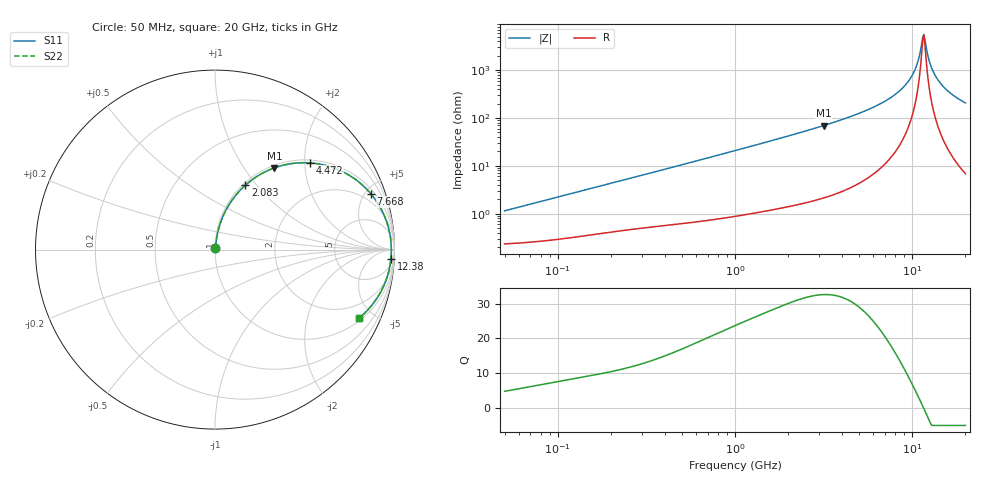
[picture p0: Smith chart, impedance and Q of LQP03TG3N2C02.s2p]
!Murata Part Number: LQP03TG3N2C02
!These Parameters are Measured in Series Mode Connection
!  o--[Z]--o
!Port1  Port2
!  o-------o
!Freq. Start=50[MHz] Stop=20[GHz], 401[Steps]
# Hz S RI R 50
!Freq.(Hz) S11(Real) S11(Imag) S21(Real) S21(Imag) S12(Real) S12(Imag) S22(Real) S22(Imag)
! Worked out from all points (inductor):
!   401 points, 50 MHz to 20 GHz, reference 50 ohm
!   read as one part in series: L = 3.56 nH near 51.52 MHz
!   highest Q = 32.6 at 3.169 GHz (marker M1), where L = 3.49 nH
!   self-resonance near 11.49 GHz
!   S11 on the Smith chart (normalised r, x): 50 MHz: 1.00, +0.02; 2.083 GHz: 1.03, +0.88; 4.472 GHz: 1.07, +2.13; 7.668 GHz: 1.31, +5.48; 12.38 GHz: 12, -33; 20 GHz: 1.14, -4.12
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5e7  0.00245 0.0112  0.9975 -0.0112  0.9975 -0.0112  0.00245 0.0112
1.364002e8  0.00425 0.0297  0.9957 -0.0297  0.9957 -0.0297  0.00425 0.0297
3.721004e8  0.0115 0.0772  0.9885 -0.0772  0.9885 -0.0772  0.0115 0.0772
1e9  0.049 0.1958  0.951 -0.1958  0.951 -0.1958  0.049 0.1958
2.083303e9  0.1695 0.3591  0.8305 -0.3591  0.8305 -0.3591  0.1695 0.3591
2.728004e9  0.2626 0.4248  0.7374 -0.4248  0.7374 -0.4248  0.2626 0.4248
3.168813e9  0.3306 0.4553  0.6694 -0.4553  0.6694 -0.4553  0.3306 0.4553
4.472136e9  0.5296 0.4831  0.4704 -0.4831  0.4704 -0.4831  0.5296 0.4831
5.944466e9  0.7184 0.4305  0.2816 -0.4305  0.2816 -0.4305  0.7184 0.4305
7.442007e9  0.8536 0.3276  0.1464 -0.3276  0.1464 -0.3276  0.8536 0.3276
7.668323e9  0.8691 0.3099  0.1309 -0.3099  0.1309 -0.3099  0.8691 0.3099
8.907419e9  0.9338 0.2098  0.0662 -0.2098  0.0662 -0.2098  0.9338 0.2098
1.004137e10  0.9673 0.1186  0.0327 -0.1186  0.0327 -0.1186  0.9673 0.1186
1.066139e10  0.977 0.0706  0.023 -0.0706  0.023 -0.0706  0.977 0.0706
1.131968e10  0.982 0.0217  0.018 -0.0217  0.018 -0.0217  0.982 0.0217
1.149051e10  0.9824 0.00938  0.0176 -0.00938  0.0176 -0.00938  0.9824 0.00938
1.183995e10  0.9824 -0.0152  0.0176 0.0152  0.0176 0.0152  0.9824 -0.0152
1.238412e10  0.9801 -0.0521  0.0199 0.0521  0.0199 0.0521  0.9801 -0.0521
1.314879e10  0.9726 -0.1007  0.0274 0.1007  0.0274 0.1007  0.9726 -0.1007
1.460232e10  0.9482 -0.1827  0.0518 0.1827  0.0518 0.1827  0.9482 -0.1827
1.670968e10  0.8971 -0.2788  0.1029 0.2788  0.1029 0.2788  0.8971 -0.2788
2e10  0.8014 -0.3826  0.1986 0.3826  0.1986 0.3826  0.8014 -0.3826
